// TwinCAT 3 PLC project Gear
// ProgramVersion: 3.1.4022.1
// libraries:
//   Tc2_MC2, * (Beckhoff Automation GmbH)
//   Tc2_Standard, * (Beckhoff Automation GmbH)
//   Tc2_System, * (Beckhoff Automation GmbH)
//   Tc3_Module, * (Beckhoff Automation GmbH)
// project tree:
//   DUTs/ State.TcDUT
//   / Gear_Status.TcTLO, GlobalTextList.TcGTLO, PlcTask.TcTTO, Visualization Manager.TcVMO, Visualization.TcVIS
//   POUs/ MAIN.TcPOU
// real-time tasks:
//   TASK PlcTask: cycle T#10ms, priority 20, ADS port 350
// motion (NC):
//   TASK NC-Task 1 SAF: cycle T#2ms, priority 4, ADS port 501
//   TASK NC-Task 1 SVB: cycle T#10ms, priority 8, ADS port 511
//   AXIS Axis_Master (id 1)
//     Dynamic: Acceleration=15000, Deceleration=15000, Jerk=63061.6
//     Velo: RefSearch=140.136926041667, RefSync=140.136926041667, SlowManual=700.684630208333, FastManual=4204.10778125, Fast=14013.6926041667, Maximum=14013.7
//     OtherSettings: AllowMotionCmdToSlave=true
//     encoder EncType=8
//       EncPara: ScaleFactorNumerator=166.4, ScaleFactorDenominator=1048576, MaxCount=#xffffffff
//     drive DrvType=9
//       DrvPara: MaxCount=#xffffffff, DriveControlDWord=#x00030100
//         Analog: VeloReferenz=15415.0618645833, VeloScale=1.02400649589962, ScaleFactorActTorque=0.1
//         TimeComp: TaskDelayCycles=1
//     controller CtrType=1
//       CtrPara: PriorControlFactor=1
//         Observer: BandWidth=20
//   AXIS Axis_Slave (id 2)
//     Dynamic: Acceleration=10000, Deceleration=10000, Jerk=63061.6
//     Velo: RefSearch=140.136926041667, RefSync=140.136926041667, SlowManual=700.684630208333, FastManual=4204.10778125, Fast=14013.6926041667, Maximum=14013.7
//     OtherSettings: AllowMotionCmdToSlave=true
//     encoder EncType=8
//       EncPara: ScaleFactorNumerator=166.4, ScaleFactorDenominator=1048576, MaxCount=#xffffffff
//     drive DrvType=9
//       DrvPara: MaxCount=#xffffffff, DriveControlDWord=#x00030100
//         Analog: VeloReferenz=15415.0618645833, VeloScale=1.02400649589962, ScaleFactorActTorque=0.1
//         TimeComp: TaskDelayCycles=1
//     controller CtrType=1
//       CtrPara: PriorControlFactor=1
//         Observer: BandWidth=20
// I/O:
//   DEVICE Device 1 (EtherCAT), AmsNetId 169.254.158.17.2.1
//     Term 1 (EK1200) [EK1200-5000 EtherCAT Power supply (2A E-Bus)]
//       Term 2 (EL1008) [EL1008 8Ch. Dig. Input 24V, 3ms]
//       Term 3 (EL2004) [EL2004 4Ch. Dig. Output 24V, 0.5A]
//       Term 4 (EL1259) [EL1259 8Ch. Dig Input 24V/8Ch. Dig. Output 24V with Multi-Time-Stamp]
//       Term 5 (EL1004) [EL1004 4Ch. Dig. Input 24V, 3ms]
//       Term 6 (EL2024) [EL2024 4Ch. Dig. Output 24V, 2A]
//       Term 7 (EL3204) [EL3204 4Ch. Ana. Input PT100 (RTD)]
//       Term 8 (EK1521) [EK1521 1 port EtherCAT junction (FX-MultiMode)]
//         Term 9 (EK1501) [EK1501 EtherCAT Coupler (2A E-Bus, FX-MultiMode, ID switch)]
//           Term 10 (EL1008) [EL1008 8Ch. Dig. Input 24V, 3ms]
//           Term 11 (EL2008) [EL2008 8Ch. Dig. Output 24V, 0.5A]
//           Term 12 (EL3255) [EL3255 5Ch. potentiometer measurement with sensor supply]
//           Term 13 (EL3064) [EL3064 4Ch. Ana. Input 0-10V]
//           Term 14 (EL3054) [EL3054 4Ch. Ana. Input 4-20mA]
//           Term 27 (EL9011) [EL9011 End Terminal]
//       Term 15 (EL6601) [EL6601 1 Port Switch (Ethernet, CoE)]
//       Term 16 (EL6731-0010) [EL6731-0010 PROFIBUS DP Slave]
//       Term 17 (EK1110) [EK1110 EtherCAT extension]
//     Term 18 (EK1100) [EK1100 EtherCAT Coupler (2A E-Bus)]
//       Term 19 (EL1004) [EL1004 4Ch. Dig. Input 24V, 3ms]
//       Term 20 (EL2004) [EL2004 4Ch. Dig. Output 24V, 0.5A]
//       Term 21 (EL6900) [EL6900, TwinSAFE PLC]
//       Term 22 (EL2904) [EL2904, 4 Ch. Safety Output 24V, 0.5A, TwinSAFE]
//         modules: Module 1 (FSOES), Module 2 (DO)
//       Term 23 (EL1904) [EL1904, 4 Ch. Safety Input 24V, TwinSAFE]
//         modules: Module 1 (FSOES)
//       Term 24 (EK1110) [EK1110 EtherCAT extension]
//     Drive 25 (AX5206-0000-0210) [AX5206-0000-0210 EtherCAT Drive (SoE, 2 Ch.)]
// variable links:
//   NC-Task 1 SAF/Axes/Axis_Master <-> Device 1 (EtherCAT)/Drive 25 (AX5206-0000-0210)
//     Drive/Inputs/In/nDataIn1 <-> AT 1/Following distance
//     Drive/Inputs/In/nDcOutputTime <-> InfoData/DcOutputShift
//     Drive/Inputs/In/nState1 <-> AT 1/Drive status word @bit 8
//     Drive/Inputs/In/nState2 <-> AT 1/Drive status word
//     Drive/Inputs/In/nState4 @bit 1 <-> WcState/InputToggle
//     Drive/Inputs/In/nState4 <-> WcState/WcState
//     Drive/Outputs/Out/nCtrl1 <-> MDT 1/Master control word @bit 8
//     Drive/Outputs/Out/nDataOut1 <-> MDT 1/Position command value
//     Enc/Inputs/In/nDataIn1 <-> AT 1/Position feedback 1 value
//     Enc/Inputs/In/nDcInputTime <-> InfoData/DcInputShift
//     Enc/Inputs/In/nState4 @bit 1 <-> WcState/InputToggle
//     Enc/Inputs/In/nState4 <-> WcState/WcState
//   NC-Task 1 SAF/Axes/Axis_Slave <-> Device 1 (EtherCAT)/Drive 25 (AX5206-0000-0210)
//     Drive/Inputs/In/nDataIn1 <-> AT 2/Following distance
//     Drive/Inputs/In/nDcOutputTime <-> InfoData/DcOutputShift
//     Drive/Inputs/In/nState1 <-> AT 2/Drive status word @bit 8
//     Drive/Inputs/In/nState2 <-> AT 2/Drive status word
//     Drive/Inputs/In/nState4 @bit 1 <-> WcState/InputToggle
//     Drive/Inputs/In/nState4 <-> WcState/WcState
//     Drive/Outputs/Out/nCtrl1 <-> MDT 2/Master control word @bit 8
//     Drive/Outputs/Out/nDataOut1 <-> MDT 2/Position command value
//     Enc/Inputs/In/nDataIn1 <-> AT 2/Position feedback 1 value
//     Enc/Inputs/In/nDcInputTime <-> InfoData/DcInputShift
//     Enc/Inputs/In/nState4 @bit 1 <-> WcState/InputToggle
//     Enc/Inputs/In/nState4 <-> WcState/WcState
//   Gear/Gear Instance <-> Device 1 (EtherCAT)/Term 1 (EK1200)/Term 2 (EL1008)
//     PlcTask Inputs/MAIN.EL1008_1 <-> Channel 1/Input
//     PlcTask Inputs/MAIN.EL1008_2 <-> Channel 2/Input
//     PlcTask Inputs/MAIN.EL1008_3 <-> Channel 3/Input
//   Gear/Gear Instance <-> Device 1 (EtherCAT)/Term 1 (EK1200)/Term 8 (EK1521)/Term 9 (EK1501)/Term 12 (EL3255)
//     PlcTask Inputs/MAIN.EL3255_1 <-> AI Standard Channel 1/Value
//   Gear/Gear Instance <-> NC-Task 1 SAF/Axes/Axis_Master
//     PlcTask Inputs/MAIN.Axis_Master.NcToPlc <-> Outputs/ToPlc
//     PlcTask Outputs/MAIN.Axis_Master.PlcToNc <-> Inputs/FromPlc
//   Gear/Gear Instance <-> NC-Task 1 SAF/Axes/Axis_Slave
//     PlcTask Inputs/MAIN.Axis_Slave.NcToPlc <-> Outputs/ToPlc
//     PlcTask Outputs/MAIN.Axis_Slave.PlcToNc <-> Inputs/FromPlc

CONFIGURATION Gear
    RESOURCE PLC ON TwinCAT3
        TASK PlcTask(INTERVAL := T#10ms, PRIORITY := 20);
        PROGRAM MAIN WITH PlcTask : MAIN;
    END_RESOURCE
END_CONFIGURATION

// ---- DUTs/State.TcDUT
TYPE State :
(
	Powering_Axes := 0,
	Calibrating_Master,
	Calibrating_Slave,
	Gearin_Axes,
	Moving_Master,
	GearOut_Axes,
	Stopping_Axes
);
END_TYPE

// ---- POUs/MAIN.TcPOU
PROGRAM MAIN
VAR
	Axis_Master			: Axis_ref;			//定义主轴
	Axis_Slave			: Axis_ref;			//定义从轴
	Master_Power		: MC_Power;			//主轴使能
	Slave_Power			: MC_Power;			//从轴使能
	Master_Calibrate	: MC_Jog;			//主轴点动
	Slave_Calibrate		: MC_Jog;			//从轴点动
	Axes_GearIn			: MC_GearInDyn;		//动态耦合
	Master_Move			: MC_MoveVelocity;	//主轴运动
	Axes_GearOut		: MC_GearOut;		//从轴解耦
	Master_Stop			: MC_Stop;			//主轴停止
	Slave_Stop			: MC_Stop;			//从轴停止

	iState				: INT:= 0;			//程序状态机
	rRatio				: LREAL:=-1;		//耦合系数
	bSwitch_1			: BOOL;				//切换耦合系数按钮1
	bSwitch_2			: BOOL;				//切换耦合系数按钮2
	bSwitch_3			: BOOL;				//切换耦合系数按钮3
	bGearIn				: BOOL;				//耦合按钮
	bStart				: BOOL;				//启动按钮
	bGearOut			: BOOL;				//解耦按钮	
	bStop				: BOOL;				//停止按钮
	
	EL1008_1	AT%I*	: BOOL;				//按钮1，正转点动
	EL1008_2	AT%I*	: BOOL;				//按钮2，反转点动
	EL1008_3	AT%I*	: BOOL;				//按钮3，切换需要点动的轴
	EL3255_1	AT%I*	: INT;				//电位器，调节主轴转速
	
END_VAR

CASE iState	OF
	Powering_Axes:							//运行程序自动使能两轴
		Master_Power.Enable			:= TRUE;
		Slave_Power.Enable			:= TRUE;
		IF Master_Power.Active AND Slave_Power.Active THEN
			iState					:= Calibrating_Master;
		END_IF
		
	Calibrating_Master:						//点动主轴,调整位置
		Master_Calibrate(
			Axis					:= Axis_Master, 
			JogForward				:= EL1008_1, 
			JogBackwards			:= EL1008_2, 
			Mode					:= 2, 
			Velocity				:= 15, 
			);
		IF EL1008_3 THEN
			iState					:= Calibrating_Slave;
		END_IF
		
	Calibrating_Slave:						//点动从轴,调整位置
		Slave_Calibrate(
			Axis					:= axis_slave,
			JogForward				:= EL1008_1,
			JogBackwards			:= EL1008_2,
			Mode					:= 2, 
			Velocity				:= 15,
			);	
		IF bGearIn THEN
			istate					:= Gearin_Axes;
		END_IF

	Gearin_Axes:							//电机转动前,执行耦合
		Axes_GearIn.Enable			:= TRUE;
		IF Axes_GearIn.InGear AND bStart THEN
			iState					:= Moving_Master;
		END_IF
		
	Moving_Master:							//主轴转动
		Master_Move.Execute			:= TRUE;
		IF Master_Move.InVelocity THEN
			Master_Move.Execute		:= FALSE;
		END_IF
		IF bGearOut THEN
			Axes_GearIn.Enable		:= FALSE;
			Master_Move.Execute		:= FALSE;
			iState					:= GearOut_Axes;
		END_IF
		
	GearOut_Axes:							//执行解耦
		Axes_GearOut.Execute		:= TRUE;
		IF Axes_GearOut.Done THEN
			Axes_GearOut.Execute	:= FALSE;	
		END_IF
		IF bStop THEN
			iState					:= Stopping_Axes;
		END_IF
		
	Stopping_Axes:							//停止转动
		Master_Stop.Execute			:= TRUE;
		Slave_Stop.Execute			:= TRUE;
		IF Master_Stop.Done AND Slave_Stop.Done THEN
			Master_Stop.Execute		:= FALSE;
			Slave_Stop.Execute		:= FALSE;
			Master_Move.Execute		:= FALSE;
			iState					:= Calibrating_Master;
		END_IF

END_CASE
Power_Axes();								//调用使能功能块
Gear_Axes();								//调用耦合解耦功能块
Move_Axes();								//调用轴运动功能块
Stop_Axes();								//调用停止功能块
Switch_Ratio();								//切换耦合系数

ACTION Gear_Axes:
Axes_GearIn(
	Master := Axis_Master,
	Slave := axis_Slave,
	GearRatio := rRatio,
	Acceleration:= 15000, 
	Deceleration:= 15000,	
	Ingear	=> 
	);
Axes_GearOut(
	Slave:= Axis_Slave, 
	Done=>  
	 );
END_ACTION

ACTION Move_Axes:
Master_Move(
	Axis	:= Axis_Master,
	Velocity:= EL3255_1/100,
	Direction	:= 3,
	InVelocity	=> 
	);
END_ACTION

ACTION Power_Axes:
Master_Power(
	Axis:= Axis_Master,  
	Enable_Positive:= TRUE, 
	Enable_Negative:= TRUE, 
	Override:= 100, 
	Active=> , 
	 );
Slave_Power(
	Axis:= Axis_Slave,  
	Enable_Positive:= TRUE, 
	Enable_Negative:= TRUE, 
	Override:= 100, 
	Active=> , 
	 );
END_ACTION

ACTION Stop_Axes:
Master_Stop(
	Axis:= Axis_Master, 
	Done=> 
	 );
Slave_Stop(
	Axis:= Axis_Slave, 
	Done=> 
	 );
END_ACTION

ACTION Switch_Ratio:
IF	bSwitch_1 THEN
	rRatio		:= -1;
ELSIF bSwitch_2 THEN
	rRatio		:= -2;
ELSIF bSwitch_3 THEN
	rRatio		:= -10;
END_IF
END_ACTION

END_PROGRAM

// ---- Gear_Status.TcTLO
TEXTLIST Gear_Status
  0 = '解耦状态'
  1 = '耦合状态'
   = ''
END_TEXTLIST

// ---- GlobalTextList.TcGTLO
TEXTLIST GlobalTextList
  180 = '%.2f'
  797 = '10:1 耦合'
  311 = '10:1 齿轮比'
  74 = '10:1耦合'
  990 = '10:1齿轮比'
  891 = '12速比'
  480 = '1:1'
  367 = '1:1 耦合'
  153 = '1:1 齿轮比'
  604 = '1:10速比'
  985 = '1:10齿轮比'
  386 = '1:1速比'
  663 = '1:1齿轮比'
  984 = '1:2速比'
  498 = '1:2齿轮比'
  667 = '1:3速比'
  607 = '2:1'
  589 = '2:1 耦合'
  100 = '2:1 齿轮比'
  747 = '2:1齿轮比'
  218 = 'Axis_Master:'
  701 = 'Axis_Master:%.2f'
  739 = 'Axis_Master:&.2f'
  109 = 'Axis_Slave:%.2f'
  766 = 'Axis_Slave:&.2f'
  840 = '主轴位置'
  947 = '主轴速度'
  272 = '从轴位置'
  523 = '从轴速度'
  475 = '位置清零'
  735 = '停止'
  567 = '启动'
  482 = '耦合'
  596 = '耦合/启动'
  952 = '耦合启动'
  370 = '耦合并启动'
  767 = '解耦'
END_TEXTLIST

// ---- Visualization.TcVIS
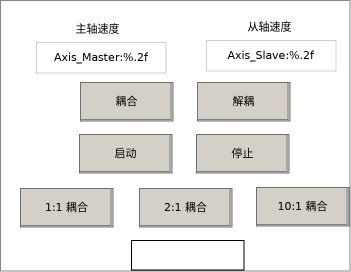
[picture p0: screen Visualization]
VISUALIZATION Visualization  // 351x272
    Label (58,14 79x30), "主轴速度"
    Textfield (36,42 130x31), "Axis_Master:%.2f", text variable: MAIN.Axis_Master.NcToPlc.ActVelo
    Label (230,12 79x30), "从轴速度"
    Textfield (206,40 130x31), "Axis_Slave:%.2f", text variable: MAIN.Axis_Slave.NcToPlc.ActVelo
    Button (79,134 93x39), "启动"
        tap MAIN.bStart
    Button (196,134 93x39), "停止"
        tap MAIN.bStop
    Button (20,188 93x39), "1:1 耦合"
        tap MAIN.bSwitch_1
    Button (139,188 93x39), "2:1 耦合"
        tap MAIN.bSwitch_2
    Button (256,187 93x39), "10:1 耦合"
        tap MAIN.bSwitch_3
    Button (80,82 93x39), "耦合"
        tap MAIN.bGearIn
    Button (197,82 93x39), "解耦"
        tap MAIN.bGearOut
    Rectangle (131,240 113x30), text list: 'Gear_Status', text index: MAIN.Axes_GearIn.InGear
END_VISUALIZATION
